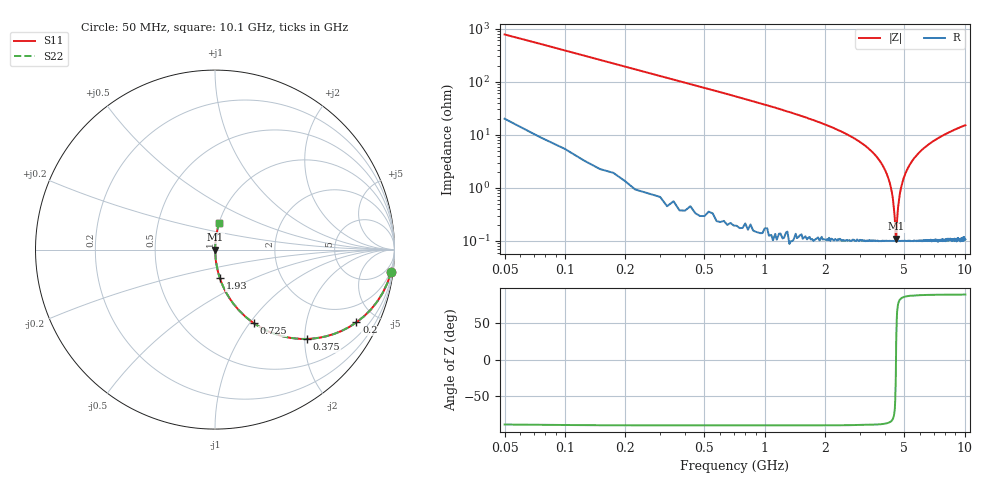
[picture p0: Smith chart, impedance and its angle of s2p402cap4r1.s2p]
! AVX Thin Film Operation		Date: April 2003
! Description: Accu-P® Series, Thin Film, SMD, RF Capacitor
! Part Number: 0402YK4R1ABW
! 50 MHz  -  10.05 GHz
! Serial Measurements
# hz S db R 50
!	S11		S21		S12		S22
!	dB	Phase	dB	Phase	dB	Phase	dB	Phase
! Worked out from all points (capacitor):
!   400 points, 50 MHz to 10.1 GHz, reference 50 ohm
!   read as one part in series: C = 4.1 pF near 100 MHz
!   lowest |Z| = 110 mohm at 4.55 GHz (marker M1)
!   series resonance near 4.54 GHz, so ESL is about 300 pH
!   S11 on the Smith chart (normalised r, x): 50 MHz: 1, -16; 200 MHz: 1.03, -3.88; 375 MHz: 1.01, -2.06; 725 MHz: 1.00, -1.04; 1.93 GHz: 1.00, -0.33; 10.1 GHz: 1.00, +0.30
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5e7  -0.10 -7.3  -17.90 81.2  -17.90 81.2  -0.10 -7.3
1e8  -0.31 -14.4  -12.10 74.8  -12.10 74.8  -0.31 -14.4
2e8  -1.05 -27.2  -6.79 62.4  -6.79 62.4  -1.05 -27.2
3.75e8  -2.91 -44.1  -3.15 45.7  -3.15 45.7  -2.91 -44.1
7.25e8  -6.71 -62.3  -1.06 27.5  -1.06 27.5  -6.71 -62.3
1.73e9  -14.50 -78.8  -0.17 10.9  -0.17 10.9  -14.50 -78.8
1.93e9  -15.80 -80.2  -0.13 9.4  -0.13 9.4  -15.80 -80.2
3.4e9  -26.00 -86.0  -0.02 2.9  -0.02 2.9  -26.00 -86.0
3.88e9  -31.30 -86.3  -0.01 1.6  -0.01 1.6  -31.30 -86.3
4.23e9  -38.20 -84.6  -0.01 0.7  -0.01 0.7  -38.20 -84.6
4.43e9  -47.10 -76.7  -0.01 0.2  -0.01 0.2  -47.10 -76.7
4.48e9  -51.70 -67.2  -0.01 0.1  -0.01 0.1  -51.70 -67.2
4.53e9  -59.10 -26.2  -0.01 0.0  -0.01 0.0  -59.10 -26.2
4.55e9  -59.20 24.2  -0.01 -0.0  -0.01 -0.0  -59.20 24.2
4.6e9  -52.00 66.6  -0.01 -0.1  -0.01 -0.1  -52.00 66.6
4.7e9  -44.30 80.2  -0.01 -0.3  -0.01 -0.3  -44.30 80.2
4.85e9  -38.90 84.3  -0.01 -0.7  -0.01 -0.7  -38.90 84.3
5.08e9  -34.30 85.9  -0.01 -1.1  -0.01 -1.1  -34.30 85.9
5.73e9  -27.90 86.3  -0.02 -2.3  -0.02 -2.3  -27.90 86.3
6.75e9  -23.20 85.2  -0.03 -4.0  -0.03 -4.0  -23.20 85.2
8.43e9  -19.00 83.0  -0.06 -6.4  -0.06 -6.4  -19.00 83.0
1.01e10  -16.50 81.0  -0.11 -8.6  -0.11 -8.6  -16.50 81.0
